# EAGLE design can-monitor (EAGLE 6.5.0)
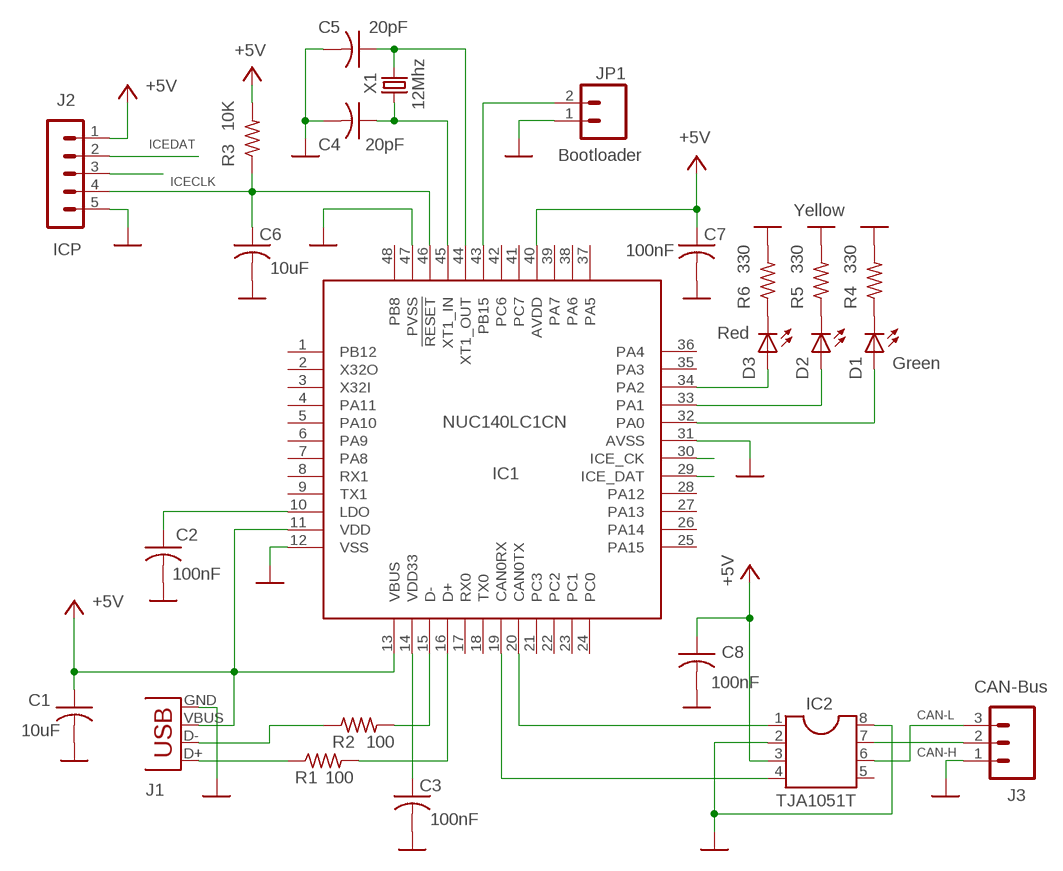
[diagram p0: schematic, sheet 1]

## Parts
C1  10uF  C-USC0805  [C0805]
C2  100nF  C-USC0805  [C0805]
C3  100nF  C-USC0805  [C0805]
C4  20pF  C-USC0805  [C0805]
C5  20pF  C-USC0805  [C0805]
C6  10uF  C-USC0805  [C0805]
C7  100nF  C-USC0805  [C0805]
C8  100nF  C-USC0805  [C0805]
D1  Green  LEDCHIPLED_0805  [CHIPLED_0805]
D2  Yellow  LEDCHIPLED_0805  [CHIPLED_0805]
D3  Red  LEDCHIPLED_0805  [CHIPLED_0805]
IC1  NUC140LC1CN  NUC140LQFP48  [LQFP48]
IC2  TJA1051T  SO-8  [SO-8]
J1  USBSMD  [USB-MINIB]
J2  MA05-1  [MA05-1]
J3  M03SCREW  [SCREWTERMINAL-3.5MM-3]
JP1  1X02  [1X02]
R1  100  R-US_R0805  [R0805]
R2  100  R-US_R0805  [R0805]
R3  10K  R-US_R0805  [R0805]
R4  330  R-US_R0805  [R0805]
R5  330  R-US_R0805  [R0805]
R6  330  R-US_R0805  [R0805]
X1  12Mhz  CRYSTALSM49  [SM49]

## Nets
+5V: C1.1 C7.1 C8.1 IC1.11(VDD) IC1.13(VBUS) IC1.40(AVDD) IC2.3 J1.VBUS J2.1 R3.2
CAN-H: IC2.7 J3.2
CAN-L: IC2.6 J3.3
CAN-RX: IC1.19(CAN0RX) IC2.4
CAN-TX: IC1.20(CAN0TX) IC2.1
D+: J1.D- R2.1
D-: J1.D+ R1.1
GND: C1.2 C2.2 C3.2 C4.2 C5.2 C6.2 C7.2 C8.2 IC1.12(VSS) IC1.31(AVSS) IC1.47(PVSS) IC2.2 IC2.8 J1.GND J2.5 J3.1 JP1.1 R4.2 R5.2 R6.2
ICECLK: IC1.30(ICE_CK) J2.3
ICEDAT: IC1.29(ICE_DAT) J2.2
N$3: IC1.43(PB15) JP1.2
N$4: D1.C R4.1
N$5: D2.C R5.1
N$6: D3.A IC1.34(PA2)
N$7: C4.1 IC1.45(XT1_IN) X1.1
N$8: D1.A IC1.32(PA0)
N$9: IC1.15(D-) R2.2
N$10: C3.1 IC1.14(VDD33)
N$11: C6.1 IC1.46(!RESET) J2.4 R3.1
N$12: C2.1 IC1.10(LDO)
N$13: IC1.16(D+) R1.2
N$14: D3.C R6.1
N$15: D2.A IC1.33(PA1)
N$16: C5.1 IC1.44(XT1_OUT) X1.2
Unconnected: IC1.1(PB12) IC1.2(X32O) IC1.3(X32I) IC1.4(PA11) IC1.5(PA10) IC1.6(PA9) IC1.7(PA8) IC1.8(RX1) IC1.9(TX1) IC1.17(RX0) IC1.18(TX0) IC1.21(PC3) IC1.22(PC2) IC1.23(PC1) IC1.24(PC0) IC1.25(PA15) IC1.26(PA14) IC1.27(PA13) IC1.28(PA12) IC1.35(PA3) IC1.36(PA4) IC1.37(PA5) IC1.38(PA6) IC1.39(PA7) IC1.41(PC7) IC1.42(PC6) IC1.48(PB8) IC2.5

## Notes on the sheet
- Bootloader
- ICP
- CAN-Bus
- J1

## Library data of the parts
C1-C8 = rcl:C-US: CAPACITOR, American symbol
D1-D3 = led:LED: LED
IC1 = nuvoton:NUC140LQFP48
IC2 = obddiag-net:SO-8
J1 = SparkFun:USB: USB Connectors USB-B-PTH is fully proven SKU : PRT-00139 USB-miniB is fully proven SKU : PRT-00587 USB-A-PCB is untested. USB-A-H is throughly reviewed, but untested. Spark Fun Electronics SKU : PRT-00437 USB-B-SMT is throughly reviewed, but untested. Needs silkscreen touching up. USB-A-S has not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
J2 = obddiag-net:MA05-1
J3 = SparkFun-Connectors:M03: Header 3 Standard 3-pin 0.1" header. Use with straight break away headers (SKU : PRT-00116), right angle break away headers (PRT-00553), swiss pins (PRT-00743), machine pins (PRT-00117), and female headers (PRT-00115). Molex polarized connector foot print use with SKU : PRT-08232 with associated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
JP1 = obddiag-net:1X02
R1-R6 = rcl:R-US_: RESISTOR, American symbol
X1 = crystal:CRYSTAL: CRYSTAL; OC_FARNELL: unknown; OC_NEWARK: unknown

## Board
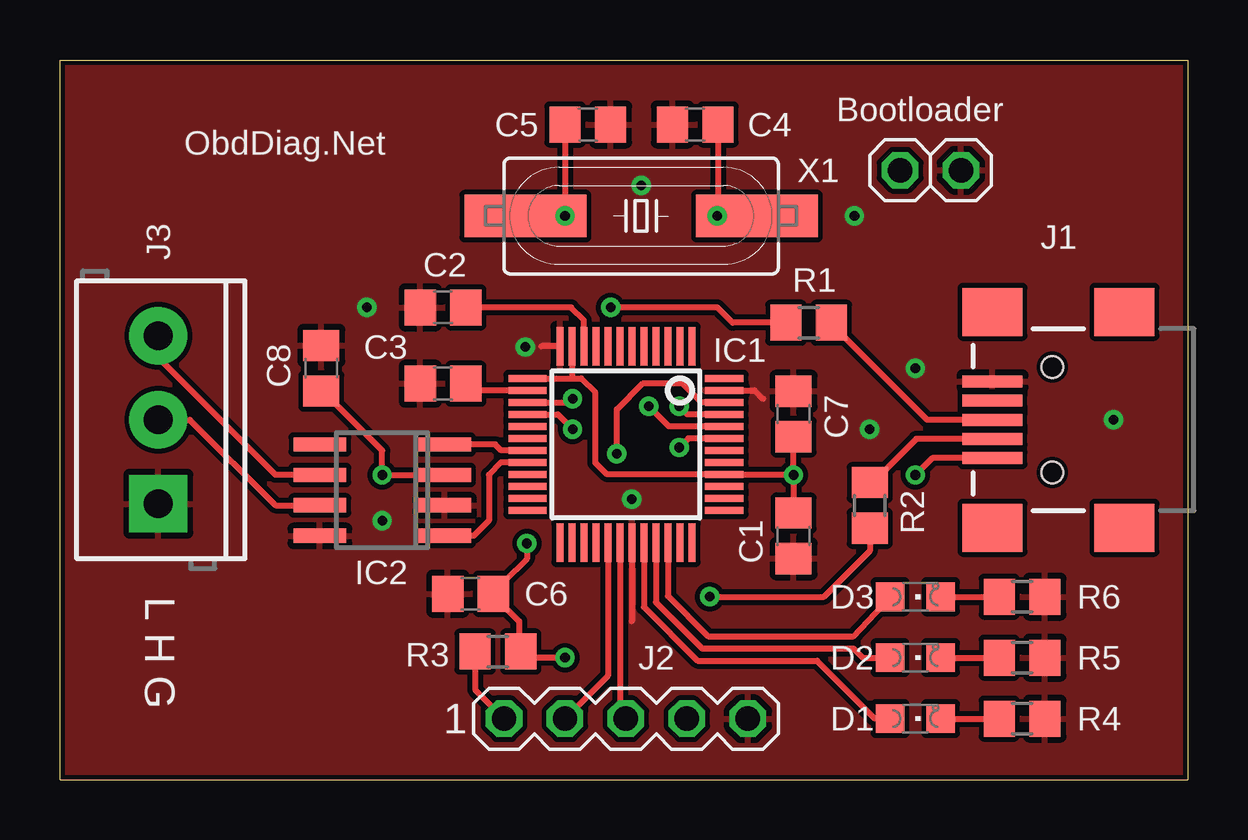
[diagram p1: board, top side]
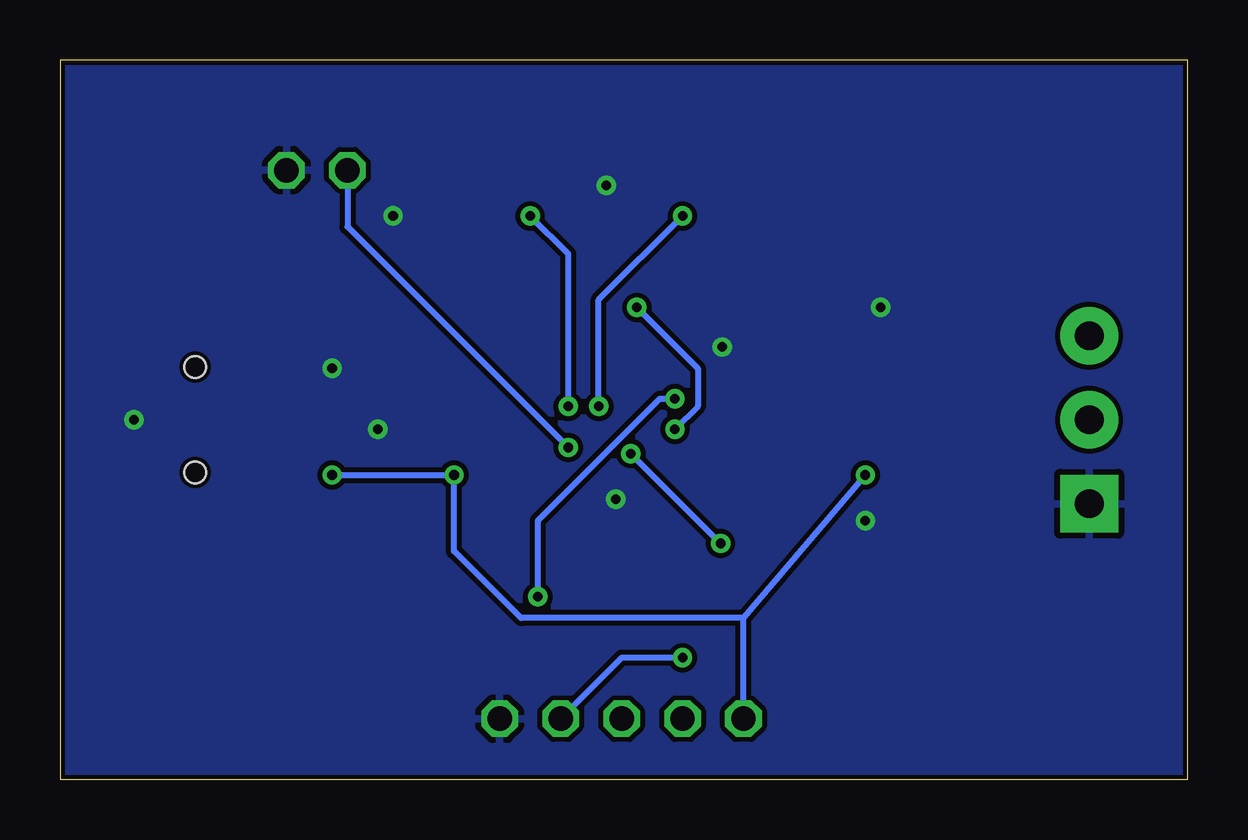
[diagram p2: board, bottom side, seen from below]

Size 47 x 30 mm. Coordinates in mm from the lower left corner, seen from the top.
Outline: 0,0 47,0 47,30 0,30 0,0
Copper layers (1*16): Top 0.035mm / dielectric 1.5mm / Bottom 0.035mm
Design rules "default *": minimum track width 10mil, minimum drill 19mil, track to track 8mil, track to pad 8mil, pad to pad 8mil, via to via 8mil, smd to smd 8mil, copper to edge 0.2mm, drill to drill 8mil, minimum pad ring 10mil, minimum via ring 8mil, stop-mask expansion 4mil, vias tented up to drill 0mil, thermal gap 10mil

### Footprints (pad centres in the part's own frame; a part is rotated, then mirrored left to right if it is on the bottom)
C0805 = smd 1.3 x 1.5: 1 -0.95,0; 2 0.95,0
CHIPLED_0805 = smd 1.2 x 1.2: A 0,-1.05; C 0,1.05
LQFP48 = smd 0.3 x 1.6: 1 -2.75,-4.1; 2 -2.25,-4.1; 3 -1.75,-4.1; 4 -1.25,-4.1; 5 -0.75,-4.1; 6 -0.25,-4.1; 7 0.25,-4.1; 8 0.75,-4.1; 9 1.25,-4.1; 10 1.75,-4.1; 11 2.25,-4.1; 12 2.75,-4.1; 25 2.75,4.1; 26 2.25,4.1; 27 1.75,4.1; 28 1.25,4.1; 29 0.75,4.1; 30 0.25,4.1; 31 -0.25,4.1; 32 -0.75,4.1; 33 -1.25,4.1; 34 -1.75,4.1; 35 -2.25,4.1; 36 -2.75,4.1 | smd 1.6 x 0.3: 13 4.1,-2.75; 14 4.1,-2.25; 15 4.1,-1.75; 16 4.1,-1.25; 17 4.1,-0.75; 18 4.1,-0.25; 19 4.1,0.25; 20 4.1,0.75; 21 4.1,1.25; 22 4.1,1.75; 23 4.1,2.25; 24 4.1,2.75; 37 -4.1,2.75; 38 -4.1,2.25; 39 -4.1,1.75; 40 -4.1,1.25; 41 -4.1,0.75; 42 -4.1,0.25; 43 -4.1,-0.25; 44 -4.1,-0.75; 45 -4.1,-1.25; 46 -4.1,-1.75; 47 -4.1,-2.25; 48 -4.1,-2.75
SO-8 = smd 0.6 x 2.2: 1 -1.905,-2.6; 2 -0.635,-2.6; 3 0.635,-2.6; 4 1.905,-2.6; 5 1.905,2.6; 6 0.635,2.6; 7 -0.635,2.6; 8 -1.905,2.6
USB-MINIB = smd 2.5 x 0.5: D+ 2.5,0; D- 2.5,0.8; GND 2.5,-1.6; ID 2.5,-0.8; VBUS 2.5,1.6 | smd 2.5 x 2: MTN1 -3,4.5; MTN2 2.5,4.5; MTN3 -3,-4.5; MTN4 2.5,-4.5 | hole 0.9: 0,2.2; 0,-2.2
MA05-1 = drill 1.016 octagon: 1 -5.08,0; 2 -2.54,0; 3 0,0; 4 2.54,0; 5 5.08,0
SCREWTERMINAL-3.5MM-3 = drill 1.2 pad 2.413 square: 1 0,0 | drill 1.2 pad 2.413: 2 3.5,0; 3 7,0
1X02 = drill 1.016 octagon: 1 -2.54,0; 2 0,0
R0805 = smd 1.3 x 1.5: 1 -0.95,0; 2 0.95,0
SM49 = smd 5.08 x 1.778: 1 -4.826,0; 2 4.826,0

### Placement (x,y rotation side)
C1  30.57,10.16 270 top
C2  15.97,19.68 180 top
C3  15.97,16.51 180 top
C4  26.48,27.3 180 top
C5  22,27.3 0 top
C6  17.11,7.75 180 top
C7  30.57,15.24 90 top
C8  10.89,17.14 90 top
D1  35.66,2.54 270 top
D2  35.66,5.08 270 top
D3  35.66,7.62 270 top
IC1  23.59,13.97 180 top
IC2  13.43,12.06 90 top
J1  41.37,15 180 top
J2  23.59,2.54 0 top
J3  4.1,11.5 90 top
JP1  35.02,25.4 180 top
R1  31.21,19.05 180 top
R2  33.75,11.43 270 top
R3  18.26,5.33 180 top
R4  40.1,2.54 0 top
R5  40.1,5.08 0 top
R6  40.1,7.62 0 top
X1  24.23,23.5 180 top

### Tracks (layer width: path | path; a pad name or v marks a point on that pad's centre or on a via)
+5V  (via drill 0.4)
  Top 0.254: v30.57,12.7 30.55,12.72 IC1.40 22.81,12.72 22.32,13.21 22.32,16.13 21.73,16.72 21.34,16.72 | v30.57,12.7 C7.1 | v30.57,12.7 C1.1 | IC1.13 21.34,16.72 | IC1.11 21.34,16.72 | IC2.3 v13.43,12.7 13.43,13.72 10.95,16.2 C8.1 | J1.VBUS 36.35,13.4 v35.66,12.7 | J2.1 17.31,3.74 R3.2
  Bottom 0.254: v35.66,12.7 v30.57,12.7 30.57,9.53 27.78,6.73 18.51,6.73 | J2.1 18.51,6.73 | v13.43,12.7 18.51,6.73
CAN-H
  Top 0.254: IC2.7 8.98,11.43 5.42,15 J3.2
CAN-L
  Top 0.254: IC2.6 8.98,12.7 4.1,17.59 J3.3
CAN-RX
  Top 0.254: IC1.19 18.39,13.72 18.14,13.97 IC2.4
CAN-TX
  Top 0.254: IC1.20 18.39,13.22 17.88,12.7 17.88,10.79 17.24,10.16 IC2.1
D+
  Top 0.254: J1.D- 35.69,14.2 34.13,12.63 34,12.63 R2.1
D-
  Top 0.254: 32.16,18.73 32.16,18.99 | R1.1 32.16,18.99 | 32.16,18.99 36.15,15 J1.D+
GND  (via drill 0.4)
  Top 0.254: IC1.47 28.96,16.22 29.3,15.88 | IC1.12 20.07,18.07 | IC1.31 23.84,6.6
  other vias: 33.11,23.5 19.4,18.03 33.75,14.61 13.43,10.79 43.91,15 23.84,11.68 35.66,17.14 12.79,19.68 24.23,24.77
  pour Bottom: 0,0 47,0 47,30 0,30
  pour Top: 0,0 47,0 47,30 0,30
ICECLK
  Top 0.254: IC1.30 23.34,2.79 J2.3
ICEDAT
  Top 0.254: IC1.29 22.84,4.33 J2.2
N$3  (via drill 0.4)
  Top 0.254: IC1.43 26.19,14.22 v25.81,13.84
  Bottom 0.254: JP1.2 35.02,23.05 v25.81,13.84
N$4
  Top 0.254: D1.C R4.1
N$5
  Top 0.254: D2.C R5.1
N$6
  Top 0.254: IC1.34 25.34,7.65 27.02,5.97 33.08,5.97 D3.A
N$7  (via drill 0.4)
  Top 0.254: IC1.45 26.15,15.22 v25.81,15.56 | C4.1 27.43,23.52 v27.4,23.5 X1.1
  Bottom 0.254: v25.81,15.56 25.81,21.91 v27.4,23.5
N$8
  Top 0.254: IC1.32 24.34,7.19 26.58,4.95 31.56,4.95 33.97,2.54 D1.A
N$9  (via drill 0.4)
  Top 0.254: IC1.15 21.21,15.72 v21.37,15.88 | v27.08,7.62 31.84,7.62 33.75,9.53 R2.2
  Bottom 0.254: v27.08,7.62 27.08,10.79 22,15.88 v21.37,15.88
N$10
  Top 0.254: IC1.14 16.57,16.22 C3.1
N$11  (via drill 0.4)
  Top 0.254: IC1.46 26.73,15.72 25.94,16.51 24.29,16.51 23.21,15.43 v23.21,13.59 | v19.46,9.84 19.46,9.21 18.51,8.26 18.51,8.19 C6.1 18.06,7.69 19.14,6.6 19.14,5.39 R3.1 19.46,5.08 v21.05,5.08
  Bottom 0.254: v19.46,9.84 v23.21,13.59 | v21.05,5.08 23.59,5.08 J2.4
N$12
  Top 0.254: IC1.10 21.84,19.15 21.3,19.68 C2.1
N$13  (via drill 0.4)
  Top 0.254: R1.2 28.04,19.05 27.4,19.68 v22.95,19.68 | IC1.16 20.75,15.22 v21.37,14.61
  Bottom 0.254: v21.37,14.61 20.41,15.56 20.41,17.14 v22.95,19.68
N$14
  Top 0.254: D3.C R6.1
N$15
  Top 0.254: IC1.33 24.84,7.39 26.77,5.46 33.08,5.46 33.46,5.08 D2.A
N$16  (via drill 0.4)
  Top 0.254: IC1.44 25.38,14.72 v24.54,15.56 | C5.1 v21.05,23.5 X1.2
  Bottom 0.254: v24.54,15.56 24.54,20 v21.05,23.5

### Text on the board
tNames: Bootloader | ObdDiag.Net | L H G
